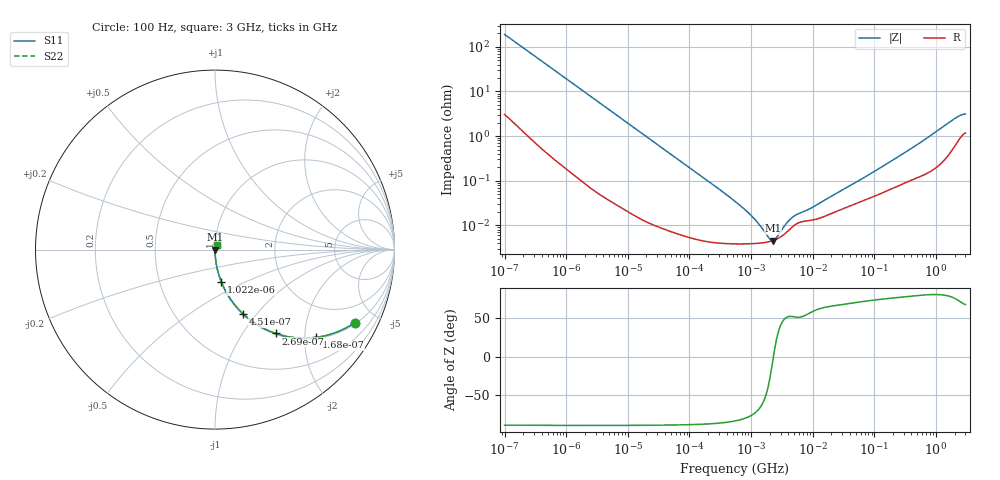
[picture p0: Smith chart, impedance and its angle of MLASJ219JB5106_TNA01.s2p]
! MLASJ219JB5106_TNA01  S-PARAMETER MODEL  ( Standard Model )
! Model Generated by TAIYO YUDEN Corporation (http://www.ty-top.com)
! Version 1.0
! TAIYO YUDEN Control No. 220601
! Copyright(c) 2009 TAIYO YUDEN CO.,LTD. All Rights Reserved.
! Product Description (link to TY-COMPAS)
! https://ds.yuden.co.jp/TYCOMPAS/or/detail?pn=MLASJ219JB5106KTNA01&u=M
! Products Name : Multilayer Ceramic Capacitors
! Characteristics :
!  Capacitance : 10 [uF] , Rated Voltage : 6.3 [V] , TCC : X5R
!  Case Size : 2.0 x 1.25 / 0.079 x 0.049 [mm/inch] , Thickness : 0.85 / 0.033 [mm/inch]
!  (Conditions: Temperature = 25 [degC] , DC Bias Voltage = 0 [V])
! External Node Assignments :
!  1  o---| |---o  2
! GND o---------o GND
! Frequency Range : 100Hz  -  3GHz  [ 401 STEP ]
# MHZ S RI R 50
! Freq[MHz].  S11 Real  S11 Imag  S21 Real  S21 Imag  S12 Real  S12 Imag  S22 Real  S22 Imag
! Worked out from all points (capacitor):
!   401 points, 100 Hz to 3 GHz, reference 50 ohm
!   read as one part in series: C = 8.37 uF near 109 Hz
!   lowest |Z| = 4.57 mohm at 2.267 MHz (marker M1)
!   series resonance near 2.301 MHz, so ESL is about 570 pH
!   S11 on the Smith chart (normalised r, x): 100 Hz: 1.06, -3.79; 168 Hz: 1.03, -2.28; 269 Hz: 1.02, -1.42; 451 Hz: 1.01, -0.85; 1.022 kHz: 1.00, -0.38; 3 GHz: 1.02, +0.06
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0.0001  0.7787 -0.4071  0.2213 0.4071  0.2213 0.4071  0.7787 -0.4071
0.000119  0.716 -0.4433  0.284 0.4433  0.284 0.4433  0.716 -0.4433
0.000168  0.5633 -0.4891  0.4367 0.4891  0.4367 0.4891  0.5633 -0.4891
0.000269  0.3378 -0.467  0.6622 0.467  0.6622 0.467  0.3378 -0.467
0.000451  0.156 -0.3577  0.844 0.3577  0.844 0.3577  0.156 -0.3577
0.000664  0.0796 -0.2658  0.9204 0.2658  0.9204 0.2658  0.0796 -0.2658
0.001022  0.036 -0.1816  0.964 0.1816  0.964 0.1816  0.036 -0.1816
0.001788  0.0125 -0.1067  0.9875 0.1067  0.9875 0.1067  0.0125 -0.1067
0.005476  0.00159 -0.0355  0.9984 0.0355  0.9984 0.0355  0.00159 -0.0355
0.031977  0.000128 -0.00614  0.9999 0.00614  0.9999 0.00614  0.000128 -0.00614
0.547723  3.85e-05 -0.000343  1 0.000343  1 0.000343  3.85e-05 -0.000343
0.842342  3.85e-05 -0.000205  1 0.000205  1 0.000205  3.85e-05 -0.000205
1.411895  4e-05 -8.86e-05  1 8.86e-05  1 8.86e-05  4e-05 -8.86e-05
2.266852  4.56e-05 -2.61e-06  1 2.61e-06  1 2.61e-06  4.56e-05 -2.61e-06
3.486191  6.37e-05 7.37e-05  0.9999 -7.37e-05  0.9999 -7.37e-05  6.37e-05 7.37e-05
5.135543  0.000102 0.00013  0.9999 -0.00013  0.9999 -0.00013  0.000102 0.00013
9.794414  0.000131 0.000215  0.9999 -0.000215  0.9999 -0.000215  0.000131 0.000215
175.1444  0.000631 0.00252  0.9994 -0.00252  0.9994 -0.00252  0.000631 0.00252
559.889  0.00129 0.00708  0.9987 -0.00708  0.9987 -0.00708  0.00129 0.00708
2036.508  0.00664 0.024  0.9934 -0.024  0.9934 -0.024  0.00664 0.024
2525.516  0.0101 0.0273  0.9899 -0.0273  0.9899 -0.0273  0.0101 0.0273
3000  0.0124 0.0284  0.9876 -0.0284  0.9876 -0.0284  0.0124 0.0284
